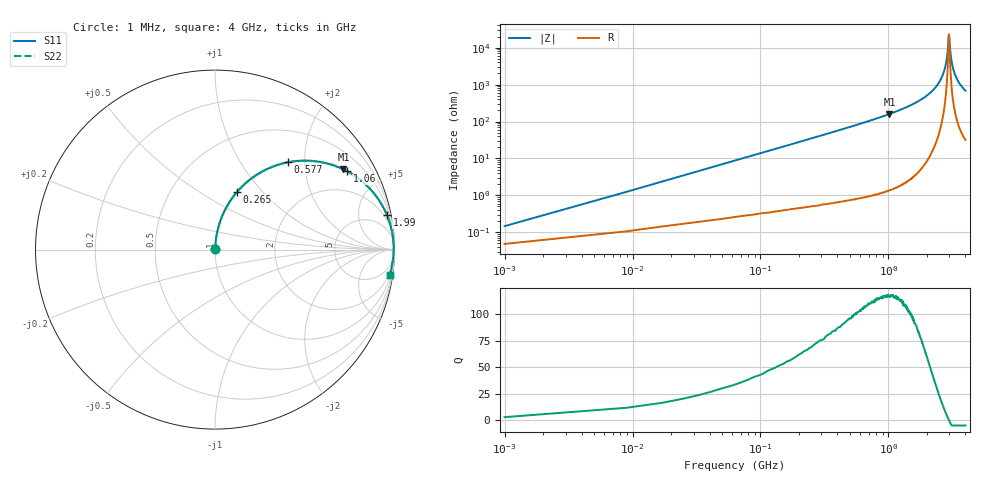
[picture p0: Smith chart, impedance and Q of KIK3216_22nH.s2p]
!version-2
!date-01.2022
!Series
# MHz S RI R 50
!Freq ReS11 ImS11 ReS21 ImS21 ReS12 ImS12 ReS22 ImS22
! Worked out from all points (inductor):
!   501 points, 1 MHz to 4 GHz, reference 50 ohm
!   read as one part in series: L = 22 nH near 17 MHz
!   highest Q = 117 at 1.02 GHz (marker M1), where L = 24.8 nH
!   self-resonance near 2.97 GHz
!   S11 on the Smith chart (normalised r, x): 1 MHz: 1.00, +0.00; 265 MHz: 1.01, +0.74; 577 MHz: 1.02, +1.66; 1.06 GHz: 1.03, +3.34; 1.99 GHz: 1, +10; 4 GHz: 2, -14
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1  0.000469 0.00138  0.9995 -0.00138  0.9995 -0.00138  0.000469 0.00138
25  0.00287 0.0344  0.9971 -0.0344  0.9971 -0.0344  0.00287 0.0344
57  0.00858 0.078  0.9914 -0.078  0.9914 -0.078  0.00858 0.078
137  0.0381 0.1819  0.9619 -0.1819  0.9619 -0.1819  0.0381 0.1819
265  0.1234 0.322  0.8766 -0.322  0.8766 -0.322  0.1234 0.322
577  0.4081 0.4866  0.5919 -0.4866  0.5919 -0.4866  0.4081 0.4866
673  0.4902 0.4953  0.5098 -0.4953  0.5098 -0.4953  0.4902 0.4953
1020  0.7153 0.447  0.2847 -0.447  0.2847 -0.447  0.7153 0.447
1060  0.7348 0.4372  0.2652 -0.4372  0.2652 -0.4372  0.7348 0.4372
1340  0.8405 0.3616  0.1595 -0.3616  0.1595 -0.3616  0.8405 0.3616
1990  0.9585 0.1913  0.0415 -0.1913  0.0415 -0.1913  0.9585 0.1913
2010  0.9601 0.1876  0.0399 -0.1876  0.0399 -0.1876  0.9601 0.1876
2420  0.9863 0.1001  0.0137 -0.1001  0.0137 -0.1001  0.9863 0.1001
2670  0.9934 0.0518  0.00658 -0.0518  0.00658 -0.0518  0.9934 0.0518
2860  0.9955 0.0197  0.00455 -0.0197  0.00455 -0.0197  0.9955 0.0197
2900  0.9956 0.013  0.0044 -0.013  0.0044 -0.013  0.9956 0.013
2950  0.9957 0.00379  0.00434 -0.00379  0.00434 -0.00379  0.9957 0.00379
2980  0.9956 -0.000114  0.00436 0.000114  0.00436 0.000114  0.9956 -0.000114
3030  0.9955 -0.00909  0.00455 0.00909  0.00455 0.00909  0.9955 -0.00909
3110  0.9949 -0.0216  0.00509 0.0216  0.00509 0.0216  0.9949 -0.0216
3340  0.9919 -0.055  0.00813 0.055  0.00813 0.055  0.9919 -0.055
4000  0.9729 -0.1408  0.0271 0.1408  0.0271 0.1408  0.9729 -0.1408
